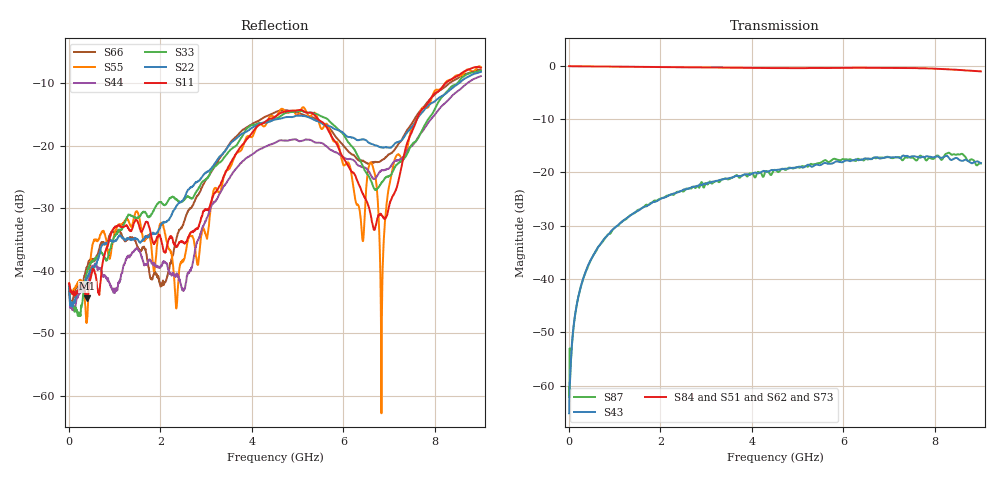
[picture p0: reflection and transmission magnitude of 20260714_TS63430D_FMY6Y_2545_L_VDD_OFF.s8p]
# GHz S DB R 50
! CMT, SN0916, 25263762, 26.7.0
! Date: 15.07.2026 14:46:01
! Data: Format
! Freq S1.1:dB/Ang S1.2:dB/Ang S1.3:dB/Ang S1.4:dB/Ang S1.5:dB/Ang S1.6:dB/Ang S1.7:dB/Ang S1.8:dB/Ang
!  S2.1:dB/Ang S2.2:dB/Ang S2.3:dB/Ang S2.4:dB/Ang S2.5:dB/Ang S2.6:dB/Ang S2.7:dB/Ang S2.8:dB/Ang
!  S3.1:dB/Ang S3.2:dB/Ang S3.3:dB/Ang S3.4:dB/Ang S3.5:dB/Ang S3.6:dB/Ang S3.7:dB/Ang S3.8:dB/Ang
!  S4.1:dB/Ang S4.2:dB/Ang S4.3:dB/Ang S4.4:dB/Ang S4.5:dB/Ang S4.6:dB/Ang S4.7:dB/Ang S4.8:dB/Ang
!  S5.1:dB/Ang S5.2:dB/Ang S5.3:dB/Ang S5.4:dB/Ang S5.5:dB/Ang S5.6:dB/Ang S5.7:dB/Ang S5.8:dB/Ang
!  S6.1:dB/Ang S6.2:dB/Ang S6.3:dB/Ang S6.4:dB/Ang S6.5:dB/Ang S6.6:dB/Ang S6.7:dB/Ang S6.8:dB/Ang
!  S7.1:dB/Ang S7.2:dB/Ang S7.3:dB/Ang S7.4:dB/Ang S7.5:dB/Ang S7.6:dB/Ang S7.7:dB/Ang S7.8:dB/Ang
!  S8.1:dB/Ang S8.2:dB/Ang S8.3:dB/Ang S8.4:dB/Ang S8.5:dB/Ang S8.6:dB/Ang S8.7:dB/Ang S8.8:dB/Ang
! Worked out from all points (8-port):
!   2001 points, 10 MHz to 9 GHz, reference 50 ohm
!   strongest paths, dB at 10 MHz, 2.257 GHz, 4.505 GHz, 6.753 GHz, 9 GHz:
!     S84: -0.1, -0.3, -0.4, -0.4, -1.0
!     S51: -0.1, -0.2, -0.5, -0.4, -1.3
!     S62: -0.1, -0.3, -0.5, -0.4, -1.2
!     S73: -0.1, -0.3, -0.5, -0.4, -1.2
!     S43: -65.2, -24.1, -19.6, -17.3, -18.2
!     S87: -61.7, -24.2, -19.5, -17.2, -18.3
!   lowest |S11| = -44.4 dB at 410.1 MHz (marker M1), VSWR 1.01, Z = 50.2 - j0.569 ohm
!   |S11| at or under -10 dB: start of sweep to 8.235 GHz
